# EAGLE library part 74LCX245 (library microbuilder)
74LCX245MTC - 5.0V Tolerant Bi-Directional Buffer Can be used to interface 5.0V logic to 2.5 or 3.3V devices Digikey: 74LCX245MTCXTR-ND Mouser: 512-74LCX245MTCX
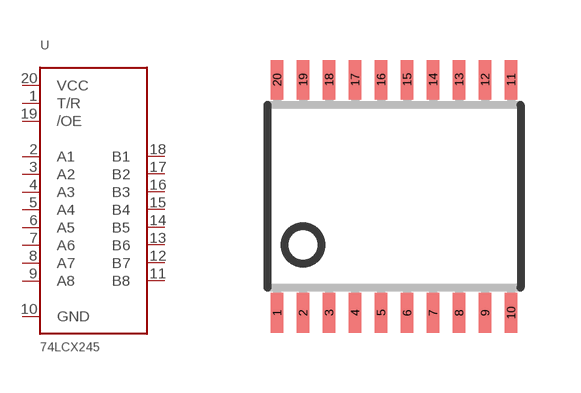
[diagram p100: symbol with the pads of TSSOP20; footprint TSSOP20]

Designator prefix U

## 74LCX245  [TSSOP20]
1  T/R
2  A1
3  A2
4  A3
5  A4
6  A5
7  A6
8  A7
9  A8
10  GND
11  B8
12  B7
13  B6
14  B5
15  B4
16  B3
17  B2
18  B1
19  /OE
20  VCC

## Footprint TSSOP20 (pad centres in mm)
smd 0.305 x 0.991: 1 -2.925,-2.918; 2 -2.275,-2.918; 3 -1.625,-2.918; 4 -0.975,-2.918; 5 -0.325,-2.918; 6 0.325,-2.918; 7 0.975,-2.918; 8 1.625,-2.918; 9 2.275,-2.918; 10 2.925,-2.918; 11 2.925,2.918; 12 2.275,2.918; 13 1.625,2.918; 14 0.975,2.918; 15 0.325,2.918; 16 -0.325,2.918; 17 -0.975,2.918; 18 -1.625,2.918; 19 -2.275,2.918; 20 -2.925,2.918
